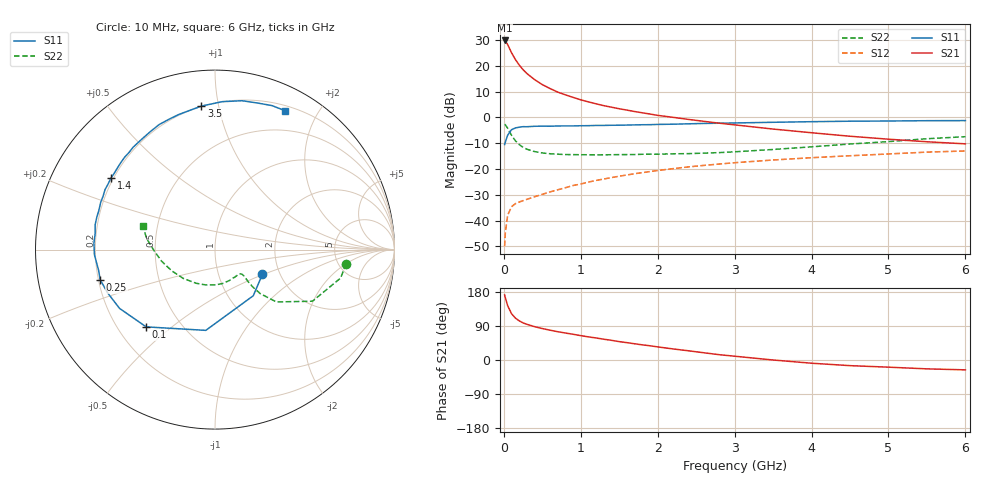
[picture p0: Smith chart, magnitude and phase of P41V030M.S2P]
! SIEMENS Small Signal Semiconductors
! BFP182
! Si NPN RF Bipolar Junction Transistor in SOT143
! VCE = 1 V  IC = 30 mA
! Common Emitter S-Parameters:  March  1996
# GHz  S  MA  R  50
!  f  S11  S21  S12  S22
! GHz  MAG  ANG  MAG  ANG  MAG  ANG  MAG  ANG
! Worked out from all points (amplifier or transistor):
!   36 points, 10 MHz to 6 GHz, reference 50 ohm
!   highest |S21| = 29.8 dB at 10 MHz (marker M1)
!   |S21| within 3 dB of that: start of sweep to 72.08 MHz
!   unconditionally stable (mu >= 1): start of sweep to 27.17 MHz; 183.9 MHz to end of sweep
!   at 250 MHz: K = 1.21, MAG = 22.6 dB, |S12| = -32.3 dB
!   at 1.4 GHz: K = 2.20, MAG = 7.4 dB, |S12| = -23.3 dB
!   at 6 GHz: K = 1.70, MAG = -3.5 dB, |S12| = -13.0 dB
!   S11 on the Smith chart (normalised r, x): 10 MHz: 1.63, -0.49; 100 MHz: 0.32, -0.41; 250 MHz: 0.21, -0.12; 1.4 GHz: 0.19, +0.30; 3.5 GHz: 0.20, +0.89; 6 GHz: 0.26, +1.59
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0.01  0.2978 -27.3  30.91 171.7  0.0032 71.8  0.7349 -6.2
0.02  0.334 -50.3  30.31 163.9  0.0059 70.3  0.7173 -12.8
0.05  0.4529 -96.5  25.68 143.1  0.0128 60.0  0.6144 -27.9
0.1  0.5766 -131.7  17.87 122.2  0.0186 43.7  0.4502 -40.4
0.15  0.6247 -148.4  13.22 110.6  0.0213 40.6  0.3524 -44.2
0.2  0.6454 -158.2  10.32 103.3  0.0229 39.9  0.2975 -44.7
0.25  0.6612 -165.3  8.383 98.0  0.0244 40.5  0.2633 -44.2
0.3  0.6589 -170.1  7.071 94.2  0.0259 42.2  0.2412 -43.4
0.4  0.6722 -177.5  5.385 87.9  0.029 45.6  0.2175 -42.3
0.5  0.6757 176.9  4.314 83.0  0.0323 47.7  0.2046 -42.3
0.6  0.6736 172.3  3.623 78.7  0.036 50.5  0.1974 -43.2
0.7  0.6818 168.4  3.092 74.7  0.0395 52.2  0.1936 -44.7
0.9  0.6828 161.5  2.44 67.9  0.0479 54.0  0.1898 -48.6
1.1  0.691 154.4  1.995 61.0  0.0558 55.0  0.1889 -53.9
1.4  0.7037 145.3  1.575 51.9  0.0682 54.7  0.189 -62.6
1.8  0.7202 134.3  1.226 40.0  0.085 52.5  0.193 -75.1
2.2  0.7378 123.8  1.002 29.2  0.1016 49.3  0.1969 -89.2
2.8  0.7706 109.2  0.772 14.0  0.1248 43.3  0.2078 -112.0
3.5  0.8033 95.4  0.594 0.0  0.1494 36.1  0.2389 -137.8
4.5  0.843 79.7  0.431 -14.9  0.1806 25.7  0.3049 -167.9
5.5  0.8629 68.4  0.337 -23.4  0.2124 15.7  0.3859 170.8
6  0.8664 63.4  0.307 -26.0  0.2236 10.1  0.4225 161.9
